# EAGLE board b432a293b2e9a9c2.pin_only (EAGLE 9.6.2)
REV: C

Size 25.4 x 17.78 mm. Coordinates in mm from the lower left corner, seen from the top.
Outline: 0,15.24 0,2.54 arc90 2.54,0 22.86,0 arc90 25.4,2.54 25.4,15.24 arc90 22.86,17.78 2.54,17.78 arc90 0,15.24
Copper layers (1*16): Top 0.035mm / dielectric 1.5mm / Bottom 0.035mm
Design rules "adafruit *": minimum track width 8mil, minimum drill 15.5mil, track to track 8mil, track to pad 8mil, pad to pad 8mil, via to via 8mil, smd to smd 8mil, copper to edge 10mil, drill to drill 8mil, minimum pad ring 10mil, minimum via ring 8mil, stop-mask expansion 2mil, vias tented up to drill 20mil, thermal gap 10mil
Net classes: 1 highpower: width 0.305 mm, drill 0.483 mm; 2 lowpower: width 0.254 mm, drill 0.483 mm

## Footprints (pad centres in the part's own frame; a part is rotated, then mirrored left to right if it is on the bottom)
0603-NO = smd 1.075 x 1: 1 -0.85,0; 2 0.85,0
0805-NO = smd 1.24 x 1.5: 1 -0.95,0; 2 0.95,0
JST_SH4 = smd 0.6 x 1.55: 1 -1.5,2.514; 2 -0.5,2.514; 3 0.5,2.514; 4 1.5,2.514 | smd 1.2 x 1.8: MT1 -2.8,-1.386; MT2 2.8,-1.386
CHIPLED_0603_NOOUTLINE = smd 0.8 x 0.8: A 0,-0.75; C 0,0.75
FIDUCIAL_1MM = smd 1 x 1: 1 0,0
1X01_OVAL = drill 1 pad 1.676 long: 1 0,0
1X05_ROUND_76 = drill 1 pad 1.93: 1 -5.08,0; 2 -2.54,0; 3 0,0; 4 2.54,0; 5 5.08,0
RESPACK_4X0603 = smd 0.45 x 0.9: 1 -1.3,-0.85; 2 -0.4,-0.85; 3 0.4,-0.85; 4 1.3,-0.85; 5 1.3,0.85; 6 0.4,0.85; 7 -0.4,0.85; 8 -1.3,0.85
SOLDERJUMPER_CLOSEDWIRE = smd 1.168 x 1.6: 1 -0.762,0; 2 0.762,0 | smd 0.635 x 0.203: WIRE 0,0
TESTPOINT_PAD_2MM = smd 2 x 2: P$1 0,0
PSOP10 = smd 0.28 x 1.45: 1 -1,-2.2; 2 -0.5,-2.2; 3 0,-2.2; 4 0.5,-2.2; 5 1,-2.2; 6 1,2.2; 7 0.5,2.2; 8 0,2.2; 9 -0.5,2.2; 10 -1,2.2
MOUNTINGHOLE_2.5_PLATED = drill 2.5 pad 3.2: P$1 0,0

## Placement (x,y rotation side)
C1  0.1uF  [0603-NO]  15.11,8.26 270 top
C3  10uF  [0805-NO]  18.29,8.26 270 top
C4  1uF  [0603-NO]  10.29,7.49 270 top
C5  1uF  [0603-NO]  16.64,8.26 270 top
CONN3  STEMMA_I2C_QT  [JST_SH4]  22.73,8.89 90 top
CONN4  STEMMA_I2C_QT  [JST_SH4]  2.67,8.89 270 top
D1  GREEN  [CHIPLED_0603_NOOUTLINE]  3.56,12.57 90 top
FID3  FIDUCIAL_1MM  [FIDUCIAL_1MM]  5.84,4.95 0 top
FID4  FIDUCIAL_1MM  [FIDUCIAL_1MM]  19.94,13.97 0 top
JP1  [1X01_OVAL]  17.78,15.24 0 top
JP2  [1X05_ROUND_76]  12.7,2.54 0 top
JP3  [1X01_OVAL]  7.62,15.24 0 top
R3  10K  [RESPACK_4X0603]  7.87,8.13 90 top
SJ1  [SOLDERJUMPER_CLOSEDWIRE]  4.19,10.79 270 bottom
TP1  [TESTPOINT_PAD_2MM]  15.24,15.88 0 top
TP2  [TESTPOINT_PAD_2MM]  10.16,15.88 0 top
TP3  [TESTPOINT_PAD_2MM]  15.24,15.88 0 bottom
TP4  [TESTPOINT_PAD_2MM]  10.16,15.88 0 bottom
U1  DRV2605LDGS  [PSOP10]  12.7,7.87 0 top
U$1  MOUNTINGHOLE2.5  [MOUNTINGHOLE_2.5_PLATED]  2.54,15.24 0 top
U$2  [SYMBOL_PLUS]  15.24,13.46 0 top
U$3  [SYMBOL_MINUS]  10.16,13.46 0 top
U$17  MOUNTINGHOLE2.5  [MOUNTINGHOLE_2.5_PLATED]  22.86,15.24 0 top
U$19  MOUNTINGHOLE2.5  [MOUNTINGHOLE_2.5_PLATED]  2.54,2.54 0 top
U$21  MOUNTINGHOLE2.5  [MOUNTINGHOLE_2.5_PLATED]  22.86,2.54 0 top
U$22  [ADAFRUIT_3.5MM]  9.14,14.1 180 top
U$25  [PCBFEAT-REV-040]  20.7,12.19 0 bottom
U$30  [STEMMAQT]  22.48,4.45 90 bottom
U$31  [STEMMAQT]  2.92,13.34 270 bottom

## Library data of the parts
C1 C3-C5 CONN3 CONN4 D1 JP1-JP3 R3 SJ1 TP1-TP4 U1 U$2 U$3 U$22 U$25 = microbuilder
FID3 FID4 = microbuilder; BOM: EXCLUDE
U$1 U$17 U$19 U$21 = adafruit_electromech; BOM: EXCLUDE
U$30 U$31 = silks

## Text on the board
tPlace: on | DRV2605L | Haptic | GND | SDA | VIN | SCL | INT
bPlace: DRV2605L | LED | I2C Haptic Driver / I2C Addr: 0x5A | VLogic/Vcc: 3-5VDC

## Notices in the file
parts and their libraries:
microbuilder: This work is placed in the public domain, and may be freely used for commercial and non-commercial work with the following conditions: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
